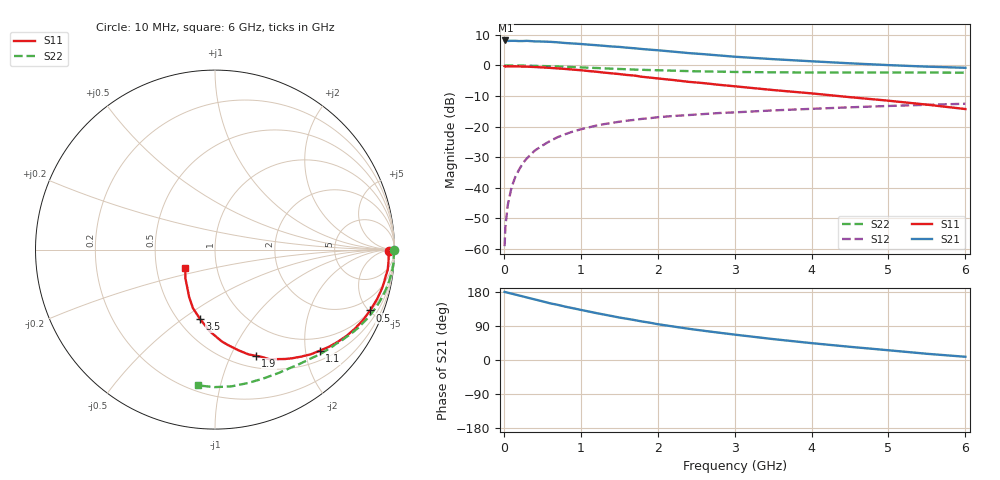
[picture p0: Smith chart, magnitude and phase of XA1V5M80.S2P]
! SIEMENS Discrete & RF Semiconductors
! BFY180
! Si NPN RF Bipolar Junction Transistor in MICRO-X
! VCE = 1.5 V  IC = 0.8 mA
! Common Emitter S-Parameters:  May  1997
# GHz  S  MA  R  50
!  f  S11  S21  S12  S22
! GHz  MAG  ANG  MAG  ANG  MAG  ANG  MAG  ANG
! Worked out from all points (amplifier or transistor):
!   36 points, 10 MHz to 6 GHz, reference 50 ohm
!   highest |S21| = 8.2 dB at 20 MHz (marker M1)
!   |S21| within 3 dB of that: start of sweep to 1.891 GHz
!   unconditionally stable (mu >= 1): 3.835 GHz to end of sweep
!   at 250 MHz: K = 0.07, MSG = 20.0 dB, |S12| = -31.9 dB
!   at 1.4 GHz: K = 0.49, MSG = 12.5 dB, |S12| = -18.8 dB
!   at 6 GHz: K = 1.07, MAG = 4.3 dB, |S12| = -12.5 dB
!   S11 on the Smith chart (normalised r, x): 10 MHz: 68, -12; 500 MHz: 1.04, -5.09; 1.1 GHz: 0.70, -2.30; 1.9 GHz: 0.63, -1.25; 3.5 GHz: 0.64, -0.59; 6 GHz: 0.70, -0.15
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0.01  0.9719 -0.3  2.533 179.8  0.0011 83.6  0.9985 -0.2
0.02  0.9563 -0.7  2.568 179.0  0.0023 92.7  0.9999 -0.6
0.05  0.9683 -2.1  2.522 177.7  0.0051 87.3  0.9974 -1.3
0.1  0.9689 -4.1  2.532 175.2  0.0101 88.6  0.9963 -2.6
0.15  0.969 -6.7  2.53 172.7  0.0151 87.0  0.9979 -4.0
0.25  0.9594 -10.9  2.513 167.7  0.0254 83.0  0.995 -6.6
0.3  0.956 -12.9  2.53 164.9  0.0302 80.5  0.991 -7.8
0.5  0.9283 -21.4  2.465 154.9  0.0488 74.5  0.979 -12.8
0.6  0.9138 -25.4  2.439 149.6  0.058 72.1  0.9705 -15.3
0.8  0.8771 -33.2  2.332 140.7  0.0751 66.0  0.9517 -20.0
1.1  0.8112 -44.0  2.195 128.1  0.0966 58.5  0.9192 -26.5
1.5  0.7236 -57.4  2.014 112.1  0.1199 49.7  0.8759 -34.2
1.9  0.6337 -69.0  1.814 98.4  0.1372 43.0  0.8416 -40.9
2  0.6135 -72.2  1.775 94.5  0.1421 41.7  0.8354 -42.5
2.2  0.5783 -76.6  1.685 88.5  0.1488 38.7  0.822 -45.7
2.4  0.5398 -81.8  1.596 82.5  0.1542 36.3  0.8085 -48.5
2.8  0.482 -89.7  1.459 72.0  0.1665 32.0  0.7915 -53.9
3.5  0.396 -102.1  1.269 55.2  0.1838 25.4  0.773 -63.0
4  0.3493 -110.5  1.171 44.5  0.195 21.2  0.7671 -69.5
4.5  0.3027 -118.3  1.085 34.8  0.2066 17.1  0.7657 -76.2
5.5  0.2283 -136.4  0.957 16.4  0.227 9.0  0.7662 -90.1
6  0.1934 -148.4  0.916 8.5  0.2363 4.7  0.7627 -97.1
